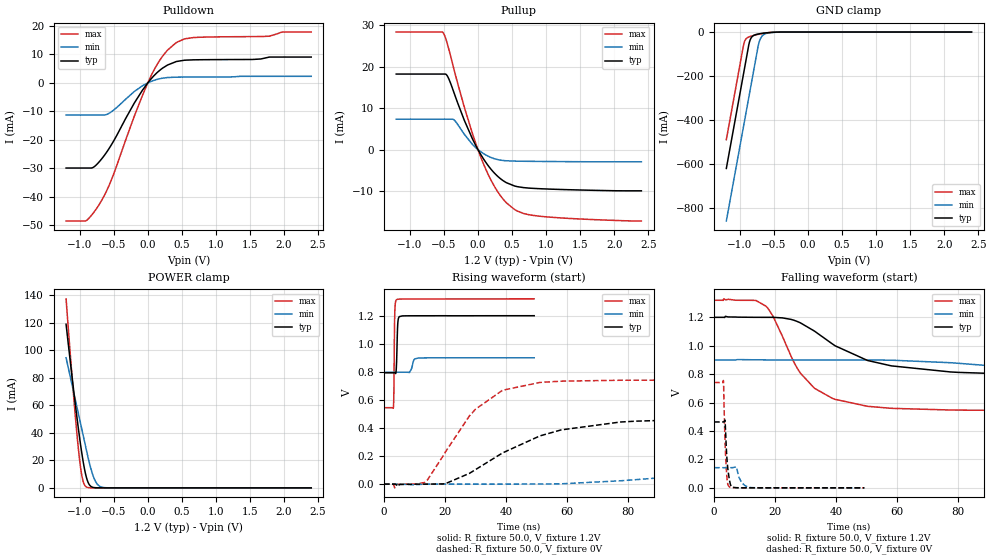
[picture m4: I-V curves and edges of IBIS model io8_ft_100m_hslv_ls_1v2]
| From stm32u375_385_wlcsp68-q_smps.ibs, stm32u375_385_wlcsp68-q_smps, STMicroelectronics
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[Model]   io8_ft_100m_hslv_ls_1v2
Model_type I/O
Polarity   Non-Inverting
Enable   Active-Low
| CAP_THRESHOLD on pad IOFT is "UDTCAPC" :
| Rising=30.0% of vddiom   Falling=70.0% of vddiom
| C_comp min and max val. don't necessarily correlate with the min and max pvt
| but are the smallest and greatest pad capacitance found.
| var   typ   min   max
C_comp   2.92725pF  2.86800pF  2.98029pF
|C_comp_pullup   1.66479pF  1.49563pF  1.80316pF
|C_comp_pulldown   1.26246pF  1.37237pF  1.17713pF
Vinl = 450.0mV
Vinh = 660.0mV
Vmeas = 600.0mV   | Reference voltage for timing measurements
Cref  = 50.0pF   | Timing specification test load capacitance value
Rref  = 1.0MOhm   | Timing specification test load resistance value
Vref  = 660.0mV   | Timing specification test load voltage
[Model Spec]
| TIME_THRESHOLD on pin ZIV11 is "CMOS" :
| Rising=50.0% of vdd   Falling=50.0% of vdd
Vinl 439.50000mV 331.50001mV 485.50000mV
Vinh 752.50000mV 552.50001mV 837.50000mV
| variable   typ   min   max
[Temperature Range] 25.0 130.0 -40.0
| variable   typ   min   max
[Voltage Range] 1.2V 900.0mV 1.32V
| variable   typ   min   max
[POWER Clamp Reference] 1.2V 900.0mV 1.32V
| variable   typ   min   max
[GND Clamp Reference] 0V 0V 0V
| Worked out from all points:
|   slope of the pulldown table from 0 to 0.18 V, typ, clamps not added: 40 ohm
|   slope of the pullup table from 0 to 0.18 V, typ, clamps not added: 40 ohm
|   GND clamp passes 1 mA (typ) near -0.50 V on its own axis
|   POWER clamp passes 1 mA (typ) near -0.83 V on its own axis
|   rising waveform, R_fixture 50.0, V_fixture 1.2V: 20-80 % time 323ps typ, 788ps min, 216ps max; typ from 0.793 V to 1.2 V
|   falling waveform, R_fixture 50.0, V_fixture 1.2V: 20-80 % time 23.1ns typ, 53.5ns min, 12.7ns max; typ from 1.2 V to 0.793 V
|   rising waveform, R_fixture 50.0, V_fixture 0V: 20-80 % time 26.4ns typ, 64.6ns min, 16.1ns max; typ from 0 V to 0.464 V
|   falling waveform, R_fixture 50.0, V_fixture 0V: 20-80 % time 939ps typ, 1.79ns min, 716ps max; typ from 0.464 V to 0 V
[POWER Clamp]
-1.2V     118.8mA    94.44mA    137.2mA
-1.09V    71.2mA     69.75mA    67.14mA
-1.02V    43.22mA    54.03mA    28.67mA
-990mV    32.26mA    47.3mA     15.78mA
-970mV    25.49mA    42.81mA    9.257mA
-940mV    16.45mA    36.08mA    3.257mA
-910mV    9.238mA    29.34mA    904.6uA
-860mV    2.387mA    18.53mA    87.46uA
-790mV    204.6uA    7.049mA    3.101uA
-730mV    21.91uA    2.041mA    176.4nA
-660mV    1.594uA    337.6uA    6.282nA
2.4V      0A         0A         0A
[GND Clamp]
-1.2V     -619mA     -857.5mA   -488.2mA
-950mV    -194mA     -432.5mA   -63.18mA
-930mV    -160mA     -398.5mA   -40.87mA
-870mV    -57.95mA   -296.5mA   -22.39mA
-840mV    -28.97mA   -245.5mA   -19.16mA
-800mV    -15.67mA   -177.5mA   -15.71mA
-730mV    -8.807mA   -59.89mA   -10.55mA
-700mV    -7.204mA   -30.66mA   -8.61mA
-660mV    -5.427mA   -13.83mA   -6.309mA
-580mV    -2.713mA   -4.125mA   -2.796mA
-380mV    -62.64uA   -240.2uA   -21.17uA
2.4V      834.9pA    121.9nA    346.5pA
| variable   typ   min   max
[Pullup Reference] 1.2V 900.0mV 1.32V
| variable   typ   min   max
[Pulldown Reference] 0V 0V 0V
[Pullup]
-1.2V     18.18mA    7.313mA    28.31mA
-510mV    18.18mA    7.313mA    28.14mA
-450mV    17.75mA    7.313mA    25.51mA
-350mV    13.63mA    7.131mA    19.22mA
-80mV     2.558mA    1.232mA    3.812mA
60mV      -1.685mA   -731.7uA   -2.583mA
180mV     -4.499mA   -1.827mA   -6.982mA
300mV     -6.594mA   -2.455mA   -10.4mA
540mV     -8.791mA   -2.785mA   -14.47mA
740mV     -9.274mA   -2.835mA   -15.67mA
1.04V     -9.521mA   -2.881mA   -16.26mA
2.4V      -9.943mA   -2.947mA   -17.22mA
[Pulldown]
-1.2V     -29.93mA   -11.33mA   -48.55mA
-910mV    -29.93mA   -11.33mA   -48.48mA
-810mV    -29.8mA    -11.33mA   -46.03mA
-710mV    -27.65mA   -11.33mA   -42.6mA
-530mV    -21.58mA   -10.08mA   -33.79mA
-200mV    -7.157mA   -3.074mA   -11.82mA
40mV      1.18mA     424.5uA    2.081mA
220mV     5.228mA    1.66mA     9.479mA
420mV     7.512mA    2.015mA    14.19mA
670mV     8.097mA    2.045mA    15.93mA
1.78V     9.043mA    2.311mA    16.4mA
2.4V      9.076mA    2.311mA    17.87mA
[Ramp]
dV/dt_r 278.13493mV/26.03012ns 85.13206mV/62.97303ns 444.65328mV/15.01869ns
dV/dt_f 244.20985mV/22.46184ns 61.52274mV/52.85652ns 465.10824mV/12.62145ns
R_load = 50.0
| Removed startup time: 0s 0s 0s  .
| Removed end time: 49.25ns.
[Rising Waveform]
R_fixture   = 50.0
V_fixture   = 1.2V
V_fixture_min = 900.0mV
V_fixture_max = 1.32V
0s        793mV      797.5mV    544.8mV
3.1ns     793mV      797.5mV    546.5mV
3.25ns    793mV      797.5mV    648.3mV
3.45ns    793.1mV    797.5mV    1.107V
3.55ns    792.9mV    797.5mV    1.219V
4.15ns    875.8mV    797.5mV    1.314V
4.5ns     1.132V     797.5mV    1.317V
5.05ns    1.194V     797.5mV    1.318V
11.05ns   1.2V       897.9mV    1.319V
49.25ns   1.2V       899.9mV    1.32V
| Removed startup time: 0s 0s 0s  .
| Removed end time: 949.25ns.
[Falling Waveform]
R_fixture   = 50.0
V_fixture   = 1.2V
V_fixture_min = 900.0mV
V_fixture_max = 1.32V
0s        1.2V       900mV      1.32V
13.55ns   1.2V       900.9mV    1.319V
17.05ns   1.2V       900.4mV    1.278V
26.95ns   1.173V     900mV      853.7mV
32.9ns    1.103V     900mV      700.8mV
39.65ns   1V         900mV      623mV
58.1ns    858.4mV    898.4mV    559.6mV
95.85ns   801.5mV    850.2mV    545.4mV
193.8ns   793mV      802.1mV    544.8mV
949.3ns   793mV      797.5mV    544.8mV
| Removed startup time: 0s 0s 0s  .
| Removed end time: 949.25ns.
[Rising Waveform]
R_fixture   = 50.0
V_fixture   = 0V
V_fixture_min = 0V
V_fixture_max = 0V
0s        4.588nV    136.5nV    3.223nV
3.5ns     19.11uV    -1.169uV   -26.61mV
13.75ns   -198.6uV   -86.26uV   18.22mV
20.15ns   3.167mV    -74.99uV   229.4mV
28ns      76.44mV    -55.5uV    485mV
38.75ns   220.5mV    77.87uV    666.9mV
58.1ns    386.4mV    2.177mV    733.6mV
96.85ns   457.7mV    56.01mV    740.8mV
213.1ns   463.4mV    137.7mV    741mV
949.3ns   463.6mV    141.9mV    741.1mV
| Removed startup time: 0s 0s 0s  .
| Removed end time: 49.25ns.
[Falling Waveform]
R_fixture   = 50.0
V_fixture   = 0V
V_fixture_min = 0V
V_fixture_max = 0V
0s        463.6mV    141.9mV    741.1mV
3.05ns    464mV      141.9mV    755.7mV
3.6ns     470.5mV    141.9mV    323mV
3.95ns    309.4mV    141.9mV    156.8mV
4.4ns     157.5mV    142mV      37.97mV
5.05ns    52.97mV    142mV      5.925mV
7.25ns    1.248mV    148.1mV    755.9uV
9.05ns    426.8uV    36.99mV    588.9uV
12.05ns   293.4uV    1.772mV    589.4uV
49.25ns   69.93uV    72.84uV    21.47uV
